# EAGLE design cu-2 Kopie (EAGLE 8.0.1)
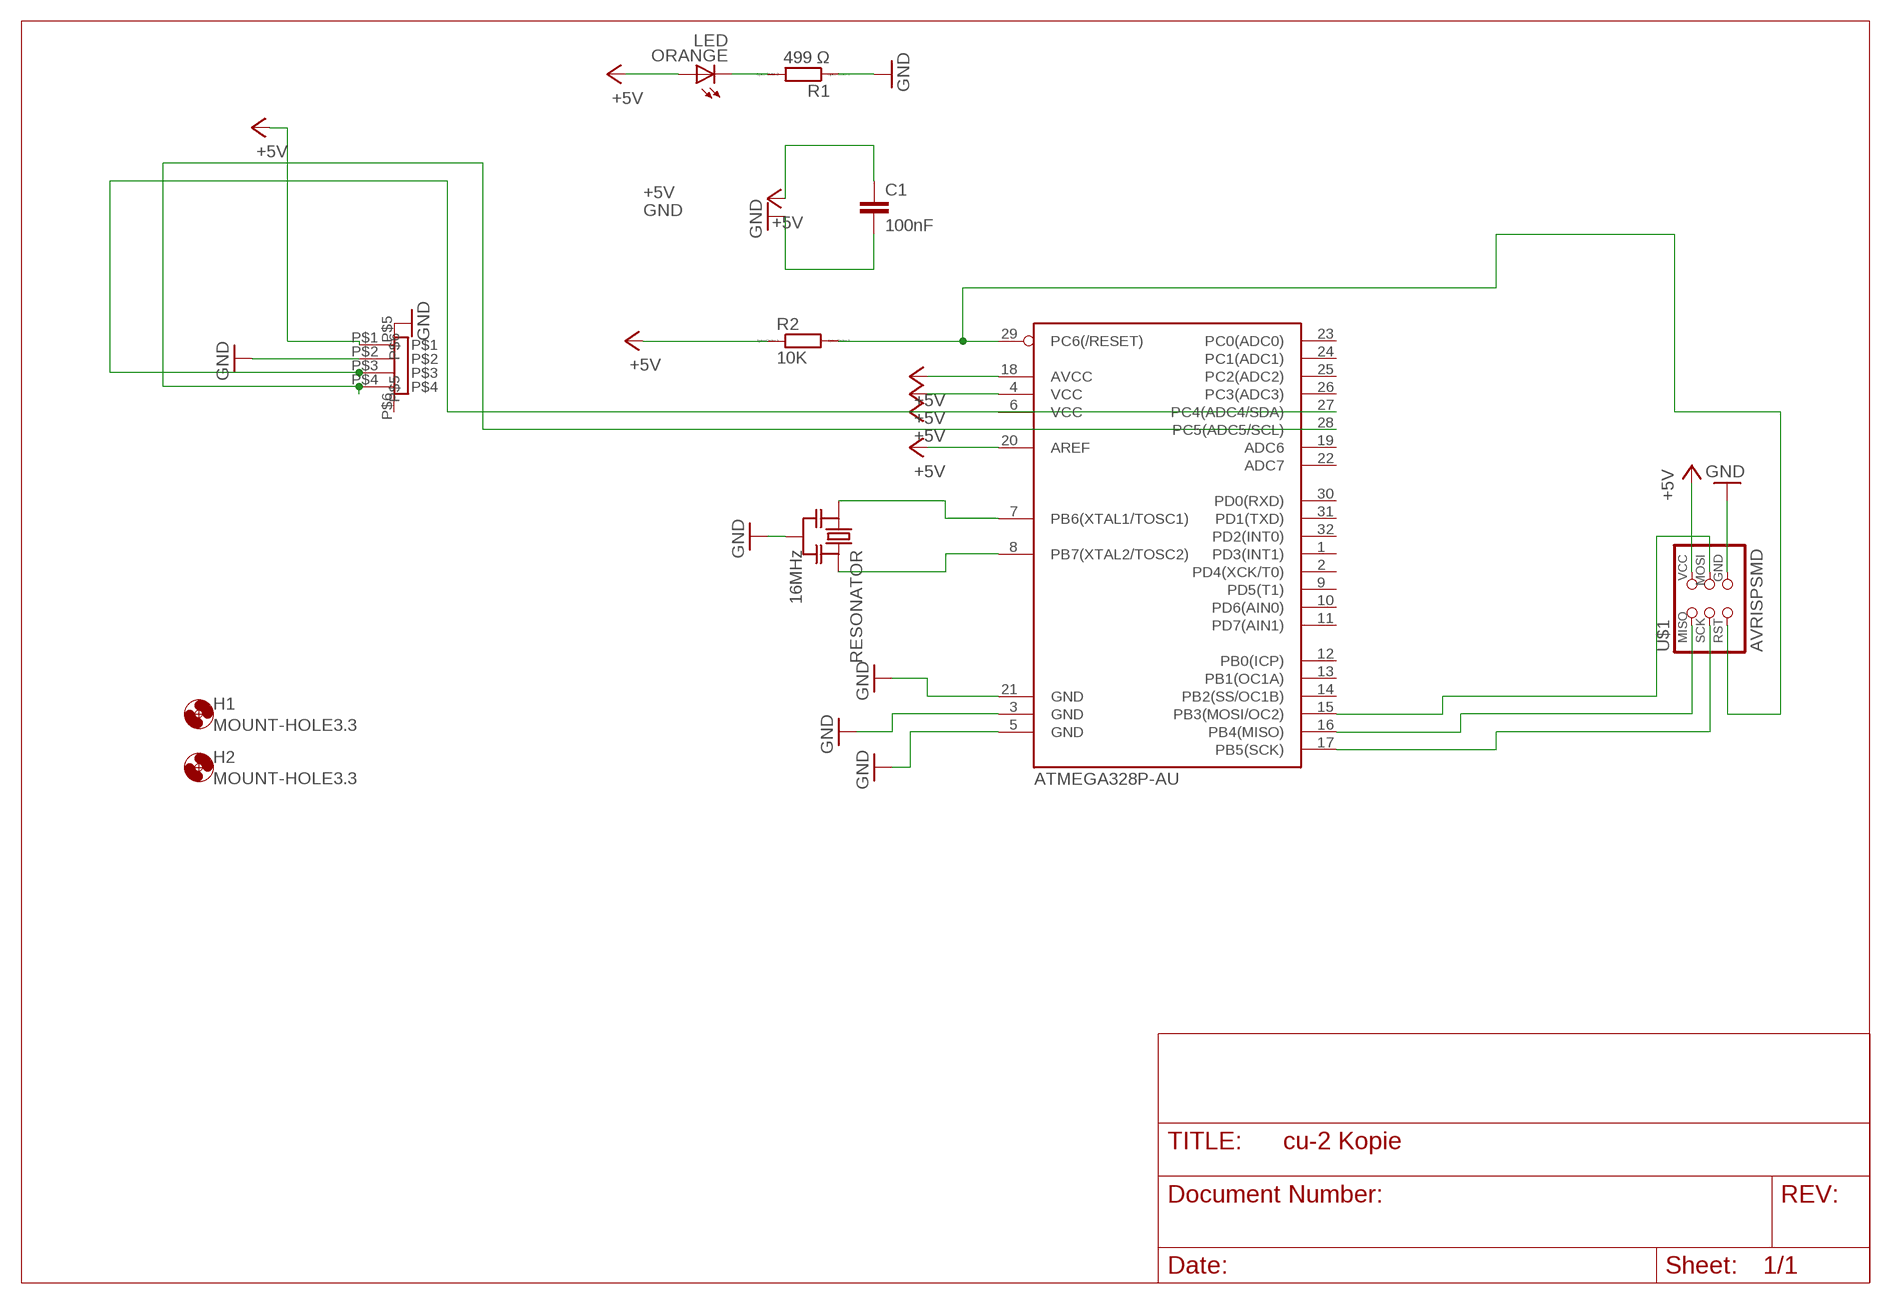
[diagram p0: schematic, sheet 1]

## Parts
ATMEGA328P-AU  ATMEGA88-THIN  [TQFP32-08THIN]
C1  100nF  C-EUC1206  [C1206]
H1  MOUNT-HOLE3.3  [3,3]
H2  MOUNT-HOLE3.3  [3,3]
ORANGE  LED  [LED1206]
R1  499 Ω  RR1206  [R1206]
R2  10K  RR1206  [R1206]
RESONATOR  16MHz  RESONATOR-MURATACSTCR_G  [RESONATOR_MURATA3]
U$1  AVRISPSMD  [2X03SMD]
U$2  PHP4_SM4  [PH4P_SM4]

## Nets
+5V: ATMEGA328P-AU.4(VCC) ATMEGA328P-AU.6(VCC) ATMEGA328P-AU.18(AVCC) ATMEGA328P-AU.20(AREF) C1.1 ORANGE.1(A) R2.1 U$1.2(VCC) U$2.P$1
GND: ATMEGA328P-AU.3(GND) ATMEGA328P-AU.5(GND) ATMEGA328P-AU.21(GND) C1.2 R1.1 RESONATOR.2 U$1.6(GND) U$2.P$2 U$2.P$5
N$6: ATMEGA328P-AU.15(PB3(MOSI/OC2)) U$1.4(MOSI)
N$19: ATMEGA328P-AU.17(PB5(SCK)) U$1.3(SCK)
N$20: ATMEGA328P-AU.16(PB4(MISO)) U$1.1(MISO)
N$24: ORANGE.2(C) R1.2
N$27: ATMEGA328P-AU.7(PB6(XTAL1/TOSC1)) RESONATOR.1
N$28: ATMEGA328P-AU.8(PB7(XTAL2/TOSC2)) RESONATOR.3
N$29: ATMEGA328P-AU.29(PC6(/RESET)) R2.2 U$1.5(RST)
SCL: ATMEGA328P-AU.28(PC5(ADC5/SCL)) U$2.P$4
SDA: ATMEGA328P-AU.27(PC4(ADC4/SDA)) U$2.P$3
Unconnected: ATMEGA328P-AU.1(PD3(INT1)) ATMEGA328P-AU.2(PD4(XCK/T0)) ATMEGA328P-AU.9(PD5(T1)) ATMEGA328P-AU.10(PD6(AIN0)) ATMEGA328P-AU.11(PD7(AIN1)) ATMEGA328P-AU.12(PB0(ICP)) ATMEGA328P-AU.13(PB1(OC1A)) ATMEGA328P-AU.14(PB2(SS/OC1B)) ATMEGA328P-AU.19(ADC6) ATMEGA328P-AU.22(ADC7) ATMEGA328P-AU.23(PC0(ADC0)) ATMEGA328P-AU.24(PC1(ADC1)) ATMEGA328P-AU.25(PC2(ADC2)) ATMEGA328P-AU.26(PC3(ADC3)) ATMEGA328P-AU.30(PD0(RXD)) ATMEGA328P-AU.31(PD1(TXD)) ATMEGA328P-AU.32(PD2(INT0)) U$2.P$6

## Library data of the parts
ATMEGA328P-AU = fab:ATMEGA88-THIN
C1 = rcl:C-EU: CAPACITOR, European symbol
H1 H2 = holes:MOUNT-HOLE: MOUNTING HOLE with drill center marker
ORANGE = fab:LED: LED
R1 R2 = eagle-ltspice:R: RESISTOR, European symbol; SPICEMODEL: NONE; SPICEPREFIX: R
RESONATOR = m-pad-2.1:RESONATOR-MURATA: Murata ceramic Resonator "ceralock" CSTCE series with built in load capacitance +- 0.5% tolerance 12.51MHz to 19.99MHz 16MHz murata part#: CSTCE16M0V53-R0 16MHz digikey part#: 490-1198-1-ND $1.33 each
U$1 = fab:AVRISP
U$2 = jst_ph_topo:PHP4_SM4

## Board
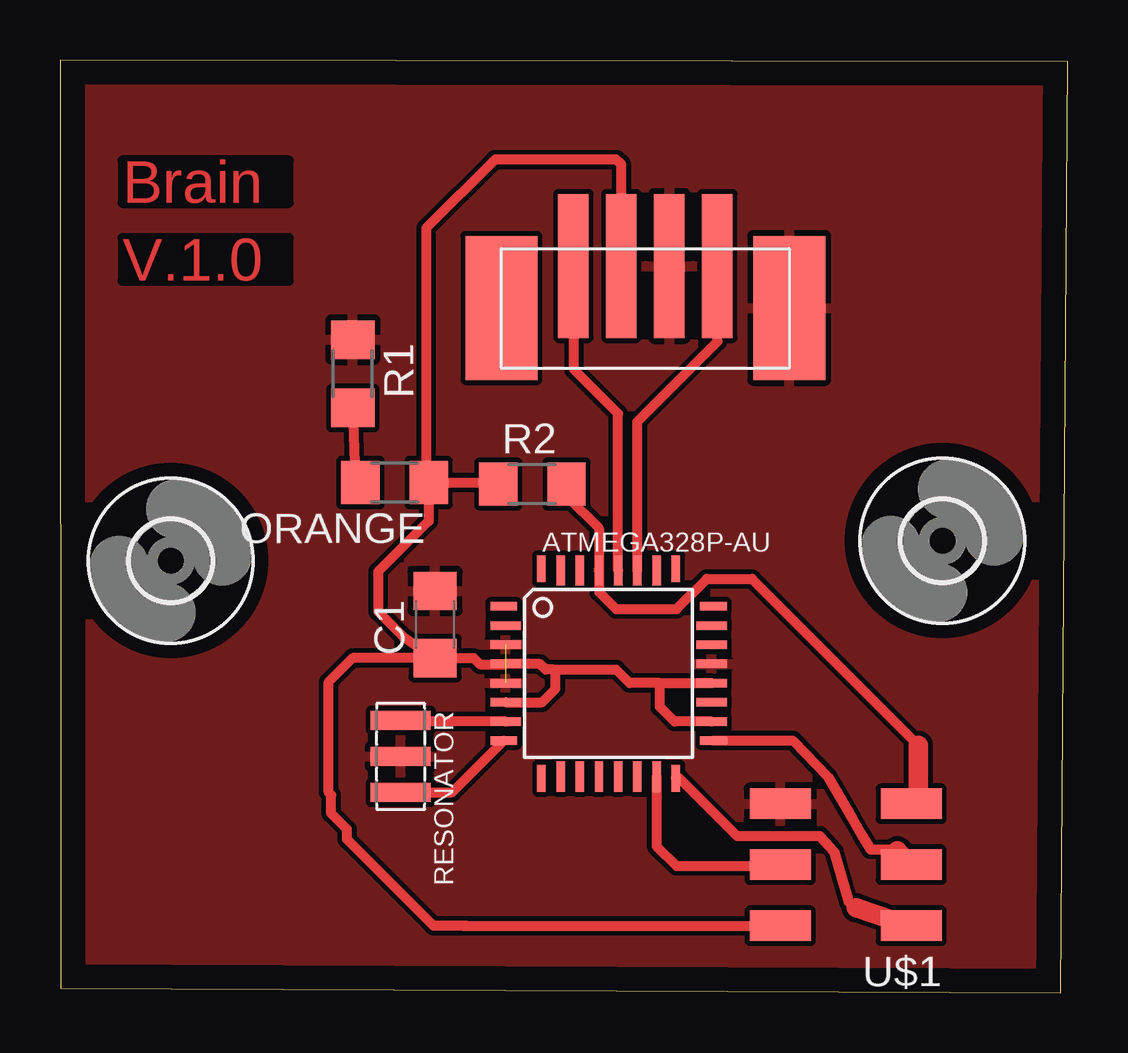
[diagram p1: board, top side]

Size 42.02 x 38.88 mm. Coordinates in mm from the lower left corner, seen from the top.
Outline: 0.03,0.19 41.71,0 42.02,38.81 0,38.88 0.03,0.19
Copper layers (1*16): Top 0.035mm / dielectric 1.5mm / Bottom 0.035mm
Design rules "default": minimum track width 10mil, minimum drill 24mil, track to track 8mil, track to pad 8mil, pad to pad 8mil, via to via 8mil, smd to smd 8mil, copper to edge 40mil, drill to drill 8mil, minimum pad ring 10mil, minimum via ring 8mil, stop-mask expansion 4mil, vias tented up to drill 0mil, thermal gap 10mil

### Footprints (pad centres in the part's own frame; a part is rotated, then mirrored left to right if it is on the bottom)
TQFP32-08THIN = smd 1.118 x 0.356: 1 -4.369,2.8; 8 -4.369,-2.8; 17 4.369,-2.8; 24 4.369,2.8 | smd 1.27 x 0.356: 2 -4.293,2; 3 -4.293,1.2; 4 -4.293,0.4; 5 -4.293,-0.4; 6 -4.293,-1.2; 7 -4.293,-2; 18 4.293,-2; 19 4.293,-1.2; 20 4.293,-0.4; 21 4.293,0.4; 22 4.293,1.2; 23 4.293,2 | smd 0.356 x 1.118: 9 -2.8,-4.369; 16 2.8,-4.369; 25 2.8,4.369; 32 -2.8,4.369 | smd 0.356 x 1.27: 10 -2,-4.293; 14 1.2,-4.293; 15 2,-4.293; 26 2,4.293; 27 1.2,4.293; 31 -2,4.293 | smd 0.35 x 1.27: 11 -1.2,-4.293; 12 -0.4,-4.293; 13 0.4,-4.293; 28 0.4,4.293; 29 -0.4,4.293; 30 -1.2,4.293
C1206 = smd 1.6 x 1.8: 1 -1.4,0; 2 1.4,0
3,3 = hole 3.3: 0,0
LED1206 = smd 1.6 x 1.803: 1 -1.422,0; 2 1.422,0
R1206 = smd 1.6 x 1.803: 1 -1.422,0; 2 1.422,0
RESONATOR_MURATA3 = smd 0.8 x 2.5: 1 -1.5,0; 2 0,0; 3 1.5,0
2X03SMD = smd 2.54 x 1.27: 1 -2.54,2.54; 2 2.92,2.54; 3 -2.54,0; 4 2.92,0; 5 -2.54,-2.54; 6 2.92,-2.54
PH4P_SM4 = smd 6 x 1.27: P$1 2,2; P$2 2,4; P$3 2,6; P$4 2,0 | smd 6 x 3: P$5 3.75,9; P$6 3.75,-3

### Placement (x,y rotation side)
ATMEGA328P-AU  22.87,13.31 0 top
C1  15.63,15.35 90 top
H1  36.78,18.84 0 top
H2  4.62,18.01 0 top
ORANGE  13.95,21.27 180 top
R1  12.2,25.8 270 top
R2  19.69,21.2 0 top
RESONATOR  14.21,9.85 270 top
U$1  32.95,5.33 180 top
U$2  21.4,32.29 270 top

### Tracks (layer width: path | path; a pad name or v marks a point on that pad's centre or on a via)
+5V
  Top 0.406: 24.98,12.91 ATMEGA328P-AU.20 | 24.98,12.91 23.74,12.91 23.18,13.47 20.56,13.47 | 20.56,13.47 20.25,13.47 20.02,13.7 ATMEGA328P-AU.4 18.56,13.69 17.51,13.69 17.25,13.95 C1.1 | ATMEGA328P-AU.18 25.61,11.31 25,11.92 25,12.89 24.98,12.91 | ATMEGA328P-AU.6 20.1,12.11 20.66,12.67 20.66,13.38 20.56,13.47 | C1.1 14.36,14.79 13.26,15.89 13.26,17.55 15.37,19.66 ORANGE.1 | U$1.2 16.93,2.79 | U$2.P$1 23.4,34.53 23.19,34.73 18.14,34.73 15.27,31.86 15.27,21.37 ORANGE.1 | ORANGE.1 18.2,21.27 R2.1 | 16.76,2.79 16.93,2.79 | C1.1 12.21,13.95 11.21,12.95 11.21,8.35 11.31,8.24 11.31,7.47 11.96,6.82 11.96,6.39 15.56,2.79 16.93,2.79
GND  (1 unrouted)
  pour Top: 43.35,40.36 -1.87,40.84 -2.04,-3.22 43.44,-3.56
N$6
  Top 0.406: ATMEGA328P-AU.15 24.87,6.11 25.7,5.28 29.97,5.28 U$1.4
N$19
  Top 0.406: ATMEGA328P-AU.17 30.55,10.51 32.02,9 33,7.29 33.42,6.57 33.78,5.97 34.85,5.97 34.91,5.91
  Top 0.813: 34.91,5.91 U$1.3
N$20
  Top 0.406: ATMEGA328P-AU.16 25.82,8.94 28.22,6.54 31.69,6.54 32.25,5.89 32.89,3.75 33.2,3.55 | 35.45,2.76 U$1.1
  Top 0.813: 33.2,3.55 35.45,2.76
N$24
  Top 0.406: R1.2 12.29,21.5 ORANGE.2
N$27
  Top 0.406: ATMEGA328P-AU.7 14.25,11.31 RESONATOR.1
N$28
  Top 0.406: RESONATOR.3 16.34,8.35 ATMEGA328P-AU.8
N$29
  Top 0.406: 35.78,10.32 28.85,17.25 26.96,17.25 25.7,15.99 23.18,15.99 22.47,16.7 ATMEGA328P-AU.29 22.46,19.36 21.11,20.71 R2.2 | 35.78,8.17 U$1.5
  Top 0.813: 35.78,10.32 35.78,8.17
SCL
  Top 0.406: ATMEGA328P-AU.28 23.27,24.14 21.43,25.98 21.43,29.62 21.4,29.65 U$2.P$4
SDA
  Top 0.406: ATMEGA328P-AU.27 24.07,23.8 27.41,27.15 27.41,30.28 U$2.P$3

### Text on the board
Top: Brain | V.1.0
